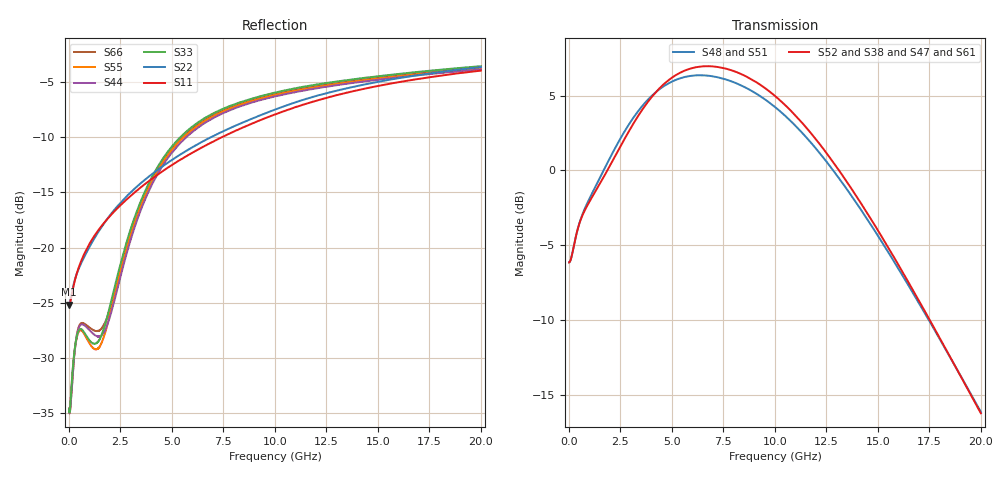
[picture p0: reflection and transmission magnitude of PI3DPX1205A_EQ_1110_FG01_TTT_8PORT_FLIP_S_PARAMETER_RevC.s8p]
! NPort=8 DATA=2000 NOISE=0 GROUPDELAY=0 COMPLEX_DATAFORMAT=POLAR
! NumOfBlock=1 NumOfParam=0
! .MODEL Smodel S TSTONEFILE=PI3DPX1205A_EQ_1110_FG01_TTT_8PORT_FLIP_S_PARAMETER_RevC.s8p TYPE=S
!  -- The above .MODEL line can be used for the S element in the netlist.
! The s parameter is extracted from the linear redriver, it is not bi-directional;
! only s(5,1)s(6,2)s(3,7)s(4,8) should be the insertion loss
!  Port definition:
!  Port1 = AIP
!  Port2 = AIN
!  Port3 = BOP
!  Port4 = BON
!  Port5 = AOP
!  Port6 = AON
!  Port7 = BIP
!  Port8 = BIN
# Hz S MA R  50
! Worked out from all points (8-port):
!   2000 points, 10 MHz to 20 GHz, reference 50 ohm
!   strongest paths, dB at 10 MHz, 5.01 GHz, 10.01 GHz, 15.01 GHz, 20 GHz:
!     S52: -6.1, 6.2, 5.0, -4.0, -16.2
!     S38: -6.1, 6.2, 5.0, -4.0, -16.2
!     S47: -6.1, 6.2, 5.0, -4.0, -16.2
!     S61: -6.1, 6.2, 5.0, -4.0, -16.2
!     S48: -6.1, 5.9, 4.2, -4.4, -16.1
!     S51: -6.1, 5.9, 4.2, -4.4, -16.1
!   lowest |S11| = -25.2 dB at 10 MHz (marker M1), VSWR 1.12, Z = 44.8 - j0.115 ohm
!   |S11| at or under -10 dB: start of sweep to 7.446 GHz
